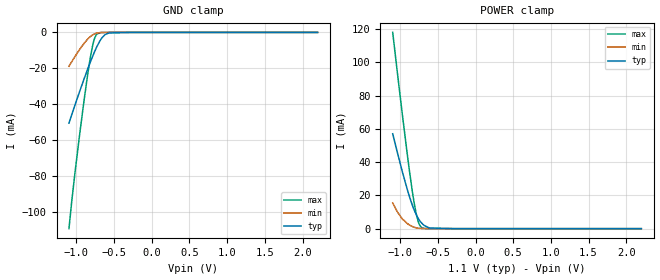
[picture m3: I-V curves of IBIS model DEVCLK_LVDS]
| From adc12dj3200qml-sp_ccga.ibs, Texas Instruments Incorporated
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[Model]   DEVCLK_LVDS
Model_type   Input
Vinl = 0.33   | Vinl & Vinh are referred to a 1.1V supply, and are an IBIS required field.
Vinh = 0.77   | However, please note that this is a differential input.
|   typ   min   max
C_comp   1.61p   1.44p   1.78p
[Voltage Range]   1.1   1.05   1.15
[Temperature Range]   25   125   -40
[Power Clamp Reference]   1.1   1.05   1.15
[GND Clamp Reference]   0   0   0
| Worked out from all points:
|   GND clamp passes 1 mA (typ) near -0.61 V on its own axis
|   POWER clamp passes 1 mA (typ) near -0.64 V on its own axis
[GND Clamp]
|   Voltage   I(typ)   I(min)   I(max)
-1.1V     -50.43mA   -18.81mA   -109.1mA
-1.064V   -45.81mA   -16.33mA   -94.18mA
-1.018V   -40.06mA   -13.26mA   -77.07mA
-905.3mV  -26.57mA   -6.435mA   -39.66mA
-852.5mV  -20.52mA   -3.789mA   -23.71mA
-819.5mV  -16.88mA   -2.45mA    -14.82mA
-789.8mV  -13.74mA   -1.512mA   -8.102mA
-760.1mV  -10.77mA   -850.6uA   -3.361mA
-730.4mV  -8.012mA   -440.1uA   -1.003mA
-664.4mV  -3.129mA   -84.69uA   -44.4uA
-568.7mV  -301.8uA   -6.98uA    -5.741uA
2.2V      0A         0A         0A
[POWER Clamp]
|   Voltage   I(typ)   I(min)   I(max)
-1.1V     57.02mA    15.46mA    118mA
-981.2mV  35.79mA    6.351mA    72.05mA
-908.6mV  23.89mA    3.168mA    45.41mA
-842.6mV  14.49mA    1.353mA    23.38mA
-809.6mV  10.6mA     769.7uA    14mA
-786.5mV  8.296mA    486uA      8.608mA
-763.4mV  6.344mA    292.3uA    4.554mA
-743.6mV  4.941mA    183.2uA    2.287mA
-710.6mV  3.087mA    80.47uA    558.7uA
-614.9mV  412.3uA    6.645uA    10.23uA
-275mV    380.1nA    58.79nA    2.316uA
2.2V      0A         0A         0A
